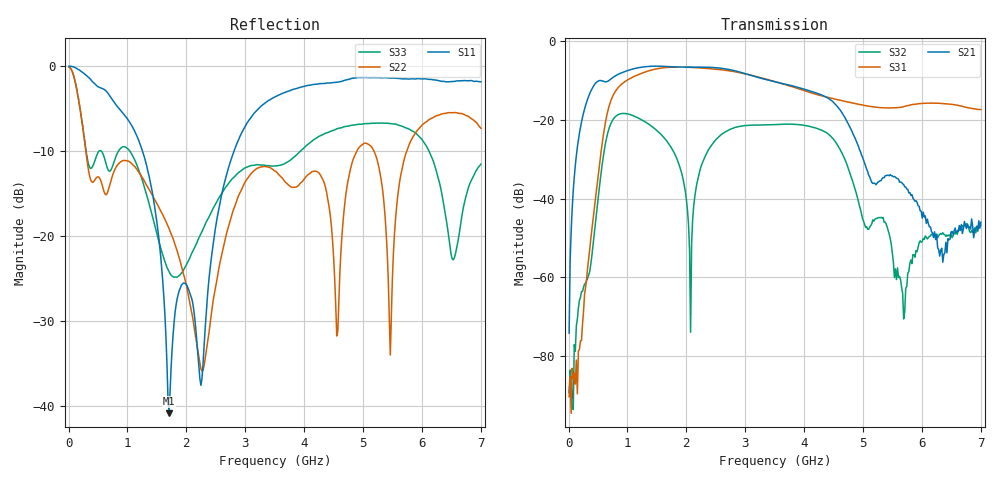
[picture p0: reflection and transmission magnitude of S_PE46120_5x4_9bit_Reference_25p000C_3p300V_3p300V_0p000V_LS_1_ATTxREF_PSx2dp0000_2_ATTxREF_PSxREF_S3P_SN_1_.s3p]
! Device ID: PE46120_5x4_9bit_Reference
! Device ID: PE46120_5x4_9bit_Reference
! File Path: z:\PE46120_5x4_9bit_Reference\MPAC_Yi\new_12port\25p000C\3p300\LS_1_ATTxREF_PSx2dp0000_2_ATTxREF_PSxREF\PE46120_5x4_9bit_Reference_25p000C_3p300V_3p300V_0p000V_LS_1_ATTxREF_PSx2dp0000_2_ATTxREF_PSxREF_S3P_SN_1_.s3p
! Serial: 1
! Lot:
! Temp: 25.000C
! VDD: 3.300
! VSS: 0.000
! Control_Hi: 3.300
! Control_Lo: 0.000
! Logic State: LS_1_ATTxREF_PSx2dp0000_2_ATTxREF_PSxREF
! Port 1: RFin
! Port 2: RFout1
! Port 3: RFout2
! ThroughPath:1-2
! IDD: -0.0005462971
! ISS: 0
! Comment:
#  Hz  S  RI  R  50
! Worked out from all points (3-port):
!   401 points, 10 MHz to 7 GHz, reference 50 ohm
!   strongest paths, dB at 10 MHz, 1.758 GHz, 3.505 GHz, 5.253 GHz, 7 GHz:
!     S21: -74.2, -6.5, -10.3, -35.8, -46.0
!     S31: -90.3, -6.6, -10.2, -16.8, -17.3
!     S32: -89.3, -27.4, -21.2, -44.9, -46.8
!   lowest |S11| = -40.9 dB at 1.705 GHz (marker M1), VSWR 1.02, Z = 50.5 - j0.756 ohm
!   |S11| at or under -10 dB: 1.257 GHz to 2.807 GHz (1.551 GHz wide, 76.3 % of centre)
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1e7  1.001 -0.0843  -0.000293 0.000271  -6.64e-05 0.000122
     -6.65e-05 0.000184  0.9888 -0.0958  3.67e-05 -8.15e-06
     -1.38e-05 2.71e-05  2.95e-05 1.72e-05  0.9879 -0.096
1.1485e8  0.5903 -0.7865  -0.0194 0.0172  -1.96e-05 1.37e-06
          -0.0196 0.0174  0.3675 -0.7178  -0.000222 1.3e-05
          -2.95e-05 3.27e-05  -0.000115 -3.91e-07  0.3639 -0.7179
3.595e8  -0.5926 -0.6102  0.1156 0.18  0.00229 0.000506
         0.1173 0.1825  -0.1805 0.1341  -0.000276 0.00132
         0.00222 0.000443  -7.56e-05 0.00118  -0.1912 0.1667
7.61425e8  -0.5766 0.24  0.2534 -0.2354  -0.203 -0.0349
           0.257 -0.2387  0.2297 -0.0524  -0.0989 0.0236
           -0.2058 -0.0357  -0.1001 0.0237  0.2402 -0.1168
1.705075e9  0.00509 -0.00748  -0.3848 0.2705  0.107 -0.4492
            -0.3898 0.2742  -0.1102 -0.0155  -0.032 0.037
            0.1082 -0.4546  -0.0321 0.0375  -0.0621 -8.2e-05
2.07205e9  -0.0445 -0.00729  0.0345 0.4622  -0.3677 -0.2765
           0.0354 0.4681  -0.0296 0.0243  -0.000123 1.73e-05
           -0.3729 -0.2794  -0.000194 -5.23e-05  -0.0759 0.00973
2.3866e9  0.0376 -0.043  0.3842 0.2553  -0.4307 0.1075
          0.3897 0.2583  -0.0269 -0.00491  -0.0273 0.0324
          -0.4363 0.1095  -0.0277 0.033  -0.0874 0.0966
3.505e9  -0.5223 -0.4075  -0.2709 -0.1324  0.3012 0.0353
         -0.275 -0.1345  0.2413 0.0192  -0.0608 -0.0618
         0.3052 0.0354  -0.0615 -0.0624  0.1789 -0.1873
5.689375e9  -0.612 0.5853  -0.00075 -0.0145  -0.1319 0.0625
            -0.00106 -0.0151  -0.1191 0.2487  -0.00125 -6.99e-05
            -0.134 0.0632  -0.000284 -8.47e-05  0.4271 0.1082
7e9  -0.1103 0.8036  0.00102 -0.00422  0.1226 0.0533
     0.00132 -0.00485  0.4171 -0.1144  -0.00396 -0.000572
     0.1249 0.0538  -0.00456 -0.000596  0.1493 0.22
